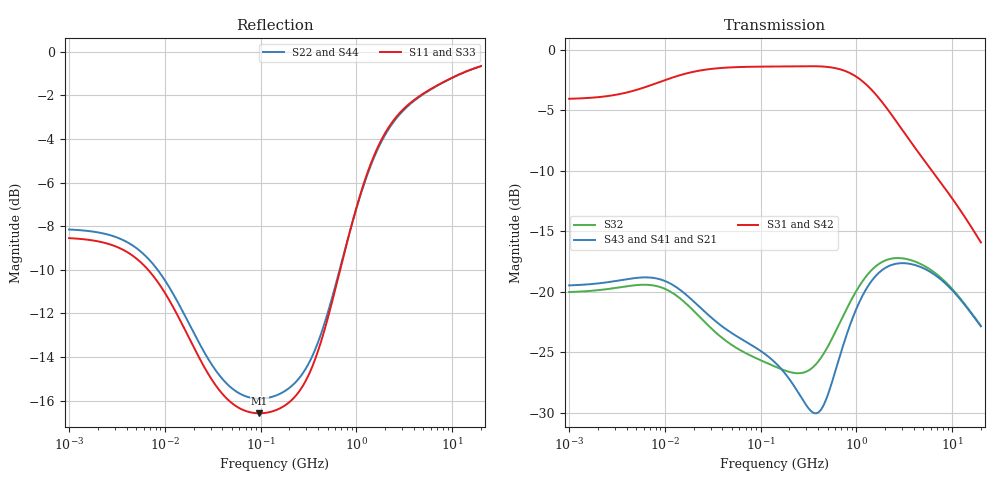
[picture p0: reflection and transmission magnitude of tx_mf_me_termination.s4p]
! Created Wed Jul 29 12:29:47 2015
# hz S db R 50
! 4 Port Network Data from SP1.SP block
! freq  dbS11  angS11  dbS12  angS12  dbS13  angS13  dbS14  angS14
!  dbS21  angS21  dbS22  angS22  dbS23  angS23  dbS24  angS24
!  dbS31  angS31  dbS32  angS32  dbS33  angS33  dbS34  angS34
!  dbS41  angS41  dbS42  angS42  dbS43  angS43  dbS44  angS44
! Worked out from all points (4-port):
!   861 points, 1 MHz to 20 GHz, reference 50 ohm
!   strongest paths, dB at 1 MHz, 11.89 MHz, 141.4 MHz, 1.682 GHz, 20 GHz:
!     S31: -4.0, -2.3, -1.4, -3.9, -15.9
!     S42: -4.3, -2.5, -1.5, -4.0, -15.9
!     S43: -19.5, -19.4, -25.9, -18.5, -22.9
!     S41: -19.5, -19.4, -25.9, -18.5, -22.9
!     S21: -19.5, -19.4, -25.9, -18.5, -22.9
!     S32: -20.0, -20.1, -26.2, -17.8, -22.8
!   lowest |S11| = -16.6 dB at 96.71 MHz (marker M1), VSWR 1.35, Z = 37.1 - j0.648 ohm
!   |S11| at or under -10 dB: 6.693 MHz to 677.7 MHz (671 MHz wide, 196 % of centre)
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1000000  -8.54 176.3  -20.03 -0.2  -4.05 2.2  -20.03 -0.2
         -19.48 0.2  -8.15 176.5  -19.48 0.2  -4.30 2.2
         -4.05 2.2  -20.03 -0.2  -8.54 176.3  -20.03 -0.2
         -19.48 0.2  -4.30 2.2  -19.48 0.2  -8.15 176.5
9230626  -10.81 158.1  -19.66 -16.4  -2.61 8.3  -19.66 -16.4
         -19.02 -14.0  -10.25 159.0  -19.02 -14.0  -2.84 8.8
         -2.61 8.3  -19.66 -16.4  -10.81 158.1  -19.66 -16.4
         -19.02 -14.0  -2.84 8.8  -19.02 -14.0  -10.25 159.0
9.671091e7  -16.58 -176.7  -25.62 -56.5  -1.39 -0.6  -25.62 -56.5
            -24.82 -44.2  -15.91 -177.3  -24.82 -44.2  -1.51 -0.5
            -1.39 -0.6  -25.62 -56.5  -16.58 -176.7  -25.62 -56.5
            -24.82 -44.2  -1.51 -0.5  -24.82 -44.2  -15.91 -177.3
3.986785e8  -13.71 -139.1  -25.80 -165.3  -1.36 -9.1  -25.80 -165.3
            -30.00 -155.6  -13.31 -142.3  -30.00 -155.6  -1.52 -9.0
            -1.36 -9.1  -25.80 -165.3  -13.71 -139.1  -25.80 -165.3
            -30.00 -155.6  -1.52 -9.0  -30.00 -155.6  -13.31 -142.3
1.136925e9  -6.35 -134.5  -19.24 87.6  -2.54 -27.4  -19.24 87.6
            -20.47 79.1  -6.40 -136.2  -20.47 79.1  -2.69 -26.8
            -2.54 -27.4  -19.24 87.6  -6.35 -134.5  -19.24 87.6
            -20.47 79.1  -2.69 -26.8  -20.47 79.1  -6.40 -136.2
2.403309e9  -3.19 -149.9  -17.25 33.0  -5.51 -40.9  -17.25 33.0
            -17.76 29.4  -3.27 -150.3  -17.76 29.4  -5.55 -40.1
            -5.51 -40.9  -17.25 33.0  -3.19 -149.9  -17.25 33.0
            -17.76 29.4  -5.55 -40.1  -17.76 29.4  -3.27 -150.3
2e10  -0.66 -171.5  -22.84 -41.2  -15.93 -58.7  -22.84 -41.2
      -22.86 -41.1  -0.66 -171.5  -22.86 -41.1  -15.92 -58.7
      -15.93 -58.7  -22.84 -41.2  -0.66 -171.5  -22.84 -41.2
      -22.86 -41.1  -15.92 -58.7  -22.86 -41.1  -0.66 -171.5
